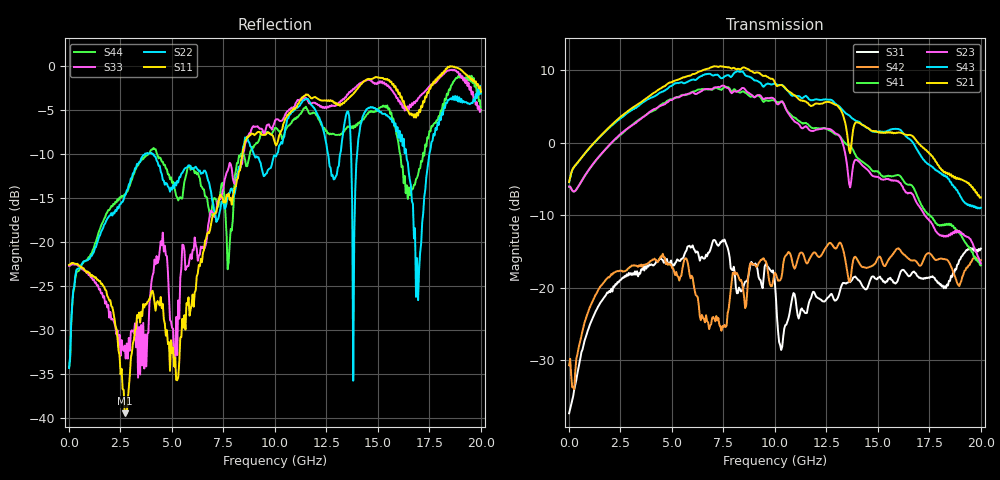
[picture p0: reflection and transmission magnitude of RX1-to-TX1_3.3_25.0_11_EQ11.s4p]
!Agilent Technologies,N5225A,MY51451112,A.09.50.13
!Agilent N5225A: A.09.50.13
!Date: Wednesday, January 31, 2018 11:05:15
!Correction: S11(Full 4 Port(1,2,3,4))
!S12(Full 4 Port(1,2,3,4))
!S13(Full 4 Port(1,2,3,4))
!S14(Full 4 Port(1,2,3,4))
!S21(Full 4 Port(1,2,3,4))
!S22(Full 4 Port(1,2,3,4))
!S23(Full 4 Port(1,2,3,4))
!S24(Full 4 Port(1,2,3,4))
!S31(Full 4 Port(1,2,3,4))
!S32(Full 4 Port(1,2,3,4))
!S33(Full 4 Port(1,2,3,4))
!S34(Full 4 Port(1,2,3,4))
!S41(Full 4 Port(1,2,3,4))
!S42(Full 4 Port(1,2,3,4))
!S43(Full 4 Port(1,2,3,4))
!S44(Full 4 Port(1,2,3,4))
!S4P File: Measurements: <S11,S12,S13,S14>,
!<S21,S22,S23,S24>,
!<S31,S32,S33,S34>,
!<S41,S42,S43,S44>:
# Hz S  RI  R 50
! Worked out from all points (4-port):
!   401 points, 10 MHz to 20 GHz, reference 50 ohm
!   strongest paths, dB at 10 MHz, 5.008 GHz, 10.01 GHz, 15 GHz, 20 GHz:
!     S21: -5.4, 8.4, 8.3, 1.5, -7.6
!     S43: -5.5, 7.9, 8.2, 1.5, -9.0
!     S23: -6.1, 5.9, 5.9, -4.7, -16.7
!     S41: -6.1, 6.0, 5.8, -3.9, -16.9
!     S42: -30.7, -17.3, -18.0, -15.9, -16.2
!     S31: -37.3, -17.2, -19.5, -18.6, -14.6
!   lowest |S11| = -39.5 dB at 2.709 GHz (marker M1), VSWR 1.02, Z = 49.1 - j0.593 ohm
!   |S11| at or under -10 dB: start of sweep to 8.426 GHz
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1e7  -0.0742 -0.00303  -0.000194 0.000469  0.0139 0.000627  -0.000272 0.000337
     0.536 0.0125  -0.0133 0.0139  -0.4976 -0.000698  0.0267 0.012
     0.0136 0.000488  -0.000415 0.000541  -0.0732 -0.00386  -4.26e-05 0.000323
     -0.4976 -0.000477  0.0266 0.012  0.5331 0.0114  -0.013 0.0146
2.70865e9  -0.00877 -0.00604  0.0158 0.00347  0.0516 0.1086  0.0175 0.000778
           1.314 -0.8934  0.1821 0.0166  -0.9619 0.7386  0.0996 0.0923
           0.0572 0.1058  0.0189 0.004  0.00694 0.0249  0.021 0.000768
           -0.8444 0.8539  0.0886 0.0946  1.07 -1.123  0.1837 -0.0341
6.956525e9  -0.0343 0.133  0.013 -0.0152  0.1405 0.0699  0.0101 -0.0268
            -3.326 0.154  0.1048 -0.1362  2.295 -0.4851  0.0269 0.0266
            0.1492 0.1372  0.0199 -0.0137  0.0273 0.1451  0.023 -0.0301
            1.873 -1.363  0.0618 -0.00596  -2.473 1.553  0.0874 -0.1347
8.6057e9  -0.00574 0.3804  0.000113 -0.00902  0.0707 0.0498  -0.00564 -0.0181
          -0.8614 3.143  -0.1199 0.3697  0.1812 -2.267  -0.0154 0.1256
          0.0949 0.0565  0.00923 -0.0166  0.0239 0.3742  -0.00906 -0.0332
          -0.8333 -2.03  -0.017 0.0733  0.82 2.768  0.2118 0.1675
1.050475e10  0.1598 0.4787  -0.0288 -0.0333  0.00745 0.019  -0.0488 -0.00306
             2.067 1.19  0.3025 0.3292  -1.689 -0.4317  0.0528 0.1909
             -0.0263 0.0485  -0.0362 -0.0305  0.2292 0.4808  -0.0539 -0.00897
             -1.681 0.4951  0.0829 0.1428  2.349 -0.1982  0.4169 -0.1083
1.42029e10  0.6695 0.4205  -0.0286 0.000274  0.00611 0.0944  -0.0124 0.0126
            0.2482 -1.314  0.4562 0.1522  0.0923 0.7021  0.1505 0.0357
            0.0178 0.1042  -0.0135 -0.00155  0.7614 0.2671  -0.0229 0.0173
            0.6409 0.3831  0.128 0.057  -1.087 -0.7946  -0.15 -0.4616
2e10  0.7116 0.0706  0.0231 0.0349  -0.0797 0.1599  0.0348 0.0207
      0.0326 0.4171  0.6935 0.0748  -0.00299 -0.1465  0.1545 0.0403
      -0.0789 0.1684  0.00625 0.0479  0.5636 -0.0246  0.0476 0.0206
      -0.1362 -0.0408  0.1478 0.046  0.3412 0.1029  -0.1515 -0.5314
